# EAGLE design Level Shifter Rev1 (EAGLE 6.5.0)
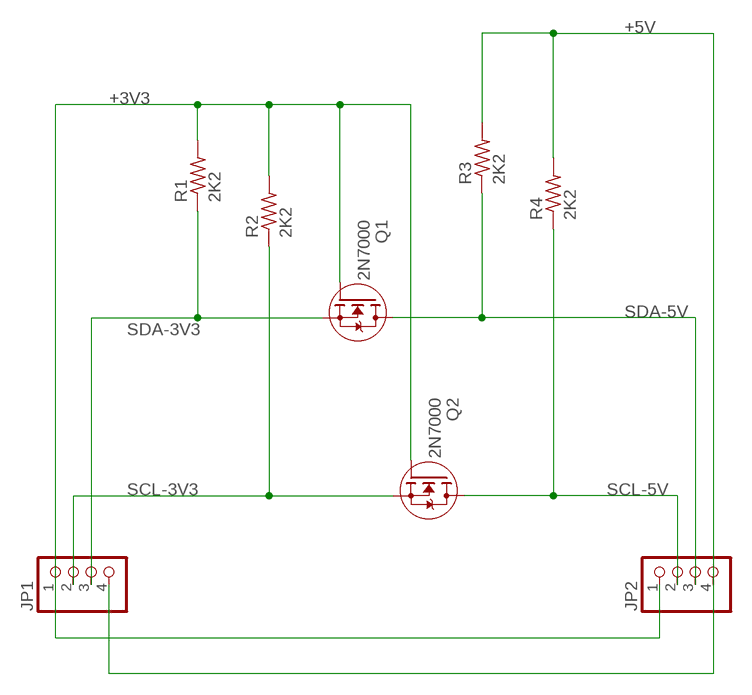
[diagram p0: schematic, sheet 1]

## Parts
JP1  PINHD-1X4  [1X04]
JP2  PINHD-1X4  [1X04]
Q1  2N7000  TO92-WIDE-STANCE  [TO92-WIDE-STANCE]
Q2  2N7000  TO92-WIDE-STANCE  [TO92-WIDE-STANCE]
R1  2K2  R-US_0204/2V  [0204V]
R2  2K2  R-US_0204/2V  [0204V]
R3  2K2  R-US_0207/2V  [0207/2V]
R4  2K2  R-US_0204/5  [0204/5]

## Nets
+3V3: JP1.1 JP2.1 Q1.2G(G) Q2.2G(G) R1.2 R2.2
+5V: JP1.4 JP2.4 R3.2 R4.2
SCL-3V3: JP1.2 Q2.1S(S) R2.1
SCL-5V: JP2.2 Q2.3D(D) R4.1
SDA-3V3: JP1.3 Q1.1S(S) R1.1
SDA-5V: JP2.3 Q1.3D(D) R3.1

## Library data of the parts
JP1 JP2 = pinhead:PINHD-1X4: PIN HEADER
Q1 Q2 = Max:TO92-WIDE-STANCE: N-Channel Mosfet, with wide stance
R1-R4 = rcl:R-US_: RESISTOR, American symbol

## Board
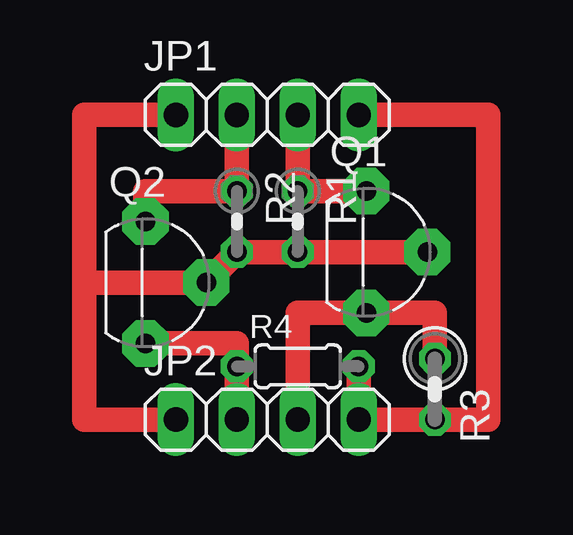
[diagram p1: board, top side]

No outline drawn. Coordinates in mm, seen from the top.
Copper layers (1*16): Top 0.035mm / dielectric 1.5mm / Bottom 0.035mm
Design rules "default": minimum track width 10mil, minimum drill 24mil, track to track 8mil, track to pad 8mil, pad to pad 8mil, via to via 8mil, smd to smd 8mil, copper to edge 40mil, drill to drill 8mil, minimum pad ring 10mil, minimum via ring 8mil, stop-mask expansion 4mil, vias tented up to drill 0mil, thermal gap 10mil

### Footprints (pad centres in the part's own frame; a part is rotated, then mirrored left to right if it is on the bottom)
1X04 = drill 1.016 long: 1 -3.81,0; 2 -1.27,0; 3 1.27,0; 4 3.81,0
TO92-WIDE-STANCE = drill 0.813 pad 1.93 octagon: 1S 0,2.54; 2G 2.54,0; 3D 0,-2.54
0204V = drill 0.813 octagon: 1 -1.27,0; 2 1.27,0
0207/2V = drill 0.813 octagon: 1 -1.27,0; 2 1.27,0
0204/5 = drill 0.813 octagon: 1 -2.54,0; 2 2.54,0

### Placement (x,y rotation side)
JP1  8.89,-20.32 0 top
JP2  8.89,-33.02 0 top
Q1  13.02,-26.04 0 top
Q2  3.81,-27.3 0 top
R1  10.16,-24.77 270 top
R2  7.62,-24.77 270 top
R3  15.88,-31.75 270 top
R4  10.16,-30.8 0 top

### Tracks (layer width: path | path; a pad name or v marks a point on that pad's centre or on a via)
+3V3
  Top 1.016: Q1.2G R1.2 R2.2 Q2.2G 1.27,-27.3 | JP2.1 1.27,-33.02 1.27,-27.3 | 1.27,-27.3 1.27,-20.32 JP1.1
+5V
  Top 1.016: JP1.4 18.1,-20.32 18.1,-33.02 R3.2 JP2.4 R4.2
SCL-3V3
  Top 1.016: JP1.2 R2.1 3.81,-23.5 Q2.1S
SCL-5V
  Top 1.016: Q2.3D 7.62,-29.84 R4.1 JP2.2
SDA-3V3
  Top 1.016: Q1.1S R1.1 JP1.3
SDA-5V
  Top 1.016: JP2.3 10.16,-28.57 Q1.3D 15.88,-28.57 R3.1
